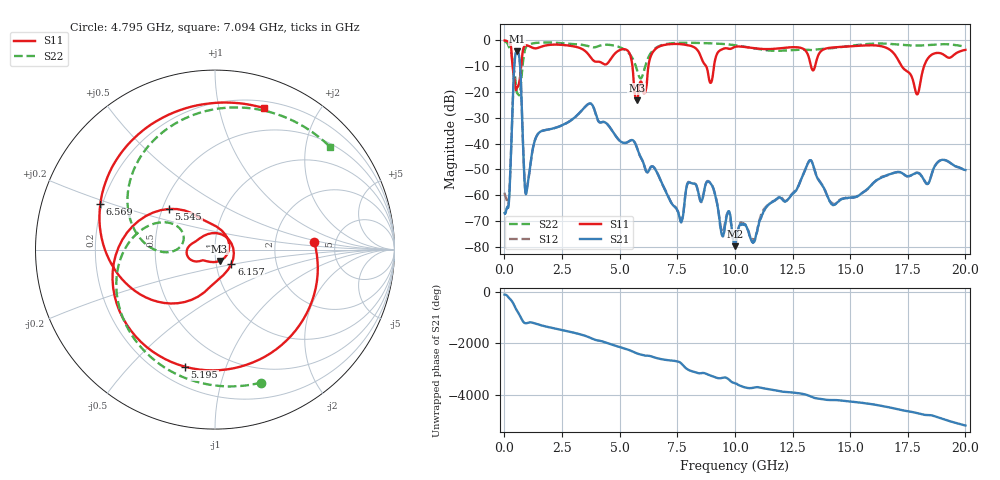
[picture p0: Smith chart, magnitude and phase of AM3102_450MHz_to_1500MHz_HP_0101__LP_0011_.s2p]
!Agilent Technologies,E8364B,MY43040894,A.07.50.67
!Agilent E8364B: A.07.50.67
!Date: Thursday, January 11, 2018 05:40:29
!Correction: S11(Full 2 Port(1,2))
!S21(Full 2 Port(1,2))
!S12(Full 2 Port(1,2))
!S22(Full 2 Port(1,2))
!S2P File: Measurements: S11, S21, S12, S22:
# Hz S  dB  R 50
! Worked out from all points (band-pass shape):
!   1601 points, 10 MHz to 20 GHz, reference 50 ohm
!   highest |S21| = -4.30 dB at 547.2 MHz (marker M1); lowest = -79.8 dB at 10.02 GHz (marker M2)
!   |S21| within 3 dB of the highest: 453.9 MHz to 658.8 MHz (205 MHz wide, 36.8 % of centre)
!   lowest |S11| = -23.3 dB at 5.745 GHz (marker M3), VSWR 1.15, Z = 52.2 - j6.63 ohm
!   |S11| at or under -10 dB: 355 MHz to 730.1 MHz (375.1 MHz wide, 69.1 % of centre); 5.555 GHz to 6.248 GHz (692.9 MHz wide, 11.7 % of centre); 17.24 GHz to 18.21 GHz (972.1 MHz wide, 5.49 % of centre)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
!   |S22| runs from -21.3 to -0.4 dB; largest |S21 - S12| = 0.0015
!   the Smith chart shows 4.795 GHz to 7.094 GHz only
!   S11 on the Smith chart (normalised r, x): 4.795 GHz: 3.43, +0.43; 5.195 GHz: 0.31, -0.73; 5.545 GHz: 0.54, +0.28; 6.157 GHz: 1.18, -0.19; 6.569 GHz: 0.19, +0.18; 7.094 GHz: 0.26, +1.37
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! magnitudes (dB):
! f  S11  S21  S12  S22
! 10 MHz  -0.1  -67.0  -59.0  -0.4
! 197.4 MHz  -0.7  -62.7  -61.3  -2.6
! 547.2 MHz  -18.3  -4.3  -4.3  -20.3
! 959.5 MHz  -2.0  -58.9  -58.6  -2.3
! 1.459 GHz  -2.9  -36.2  -36.2  -0.9
! 3.346 GHz  -3.3  -27.3  -27.3  -1.7
! 4.795 GHz  -5.1  -36.6  -36.6  -2.1
! 5.195 GHz  -3.4  -39.8  -39.8  -3.5
! 5.545 GHz  -9.3  -38.6  -38.7  -6.7
! 5.745 GHz  -23.3  -41.4  -41.4  -11.2
! 6.157 GHz  -18.3  -50.8  -50.8  -8.7
! 6.569 GHz  -3.3  -50.3  -50.3  -3.0
! 6.682 GHz  -2.6  -52.3  -52.3  -2.4
! 7.094 GHz  -1.6  -60.3  -60.1  -1.3
! 8.893 GHz  -15.6  -55.0  -54.8  -1.1
! 10.01 GHz  -2.5  -79.7  -79.4  -1.9
! 10.02 GHz  -2.5  -79.8  -79.0  -1.9
! 13.34 GHz  -11.1  -47.1  -47.1  -3.8
! 14.27 GHz  -2.8  -63.9  -63.4  -3.0
! 16.68 GHz  -3.4  -52.0  -52.1  -1.4
! 17.9 GHz  -21.0  -51.4  -51.3  -2.0
! 20 GHz  -3.7  -50.3  -50.2  -2.4
